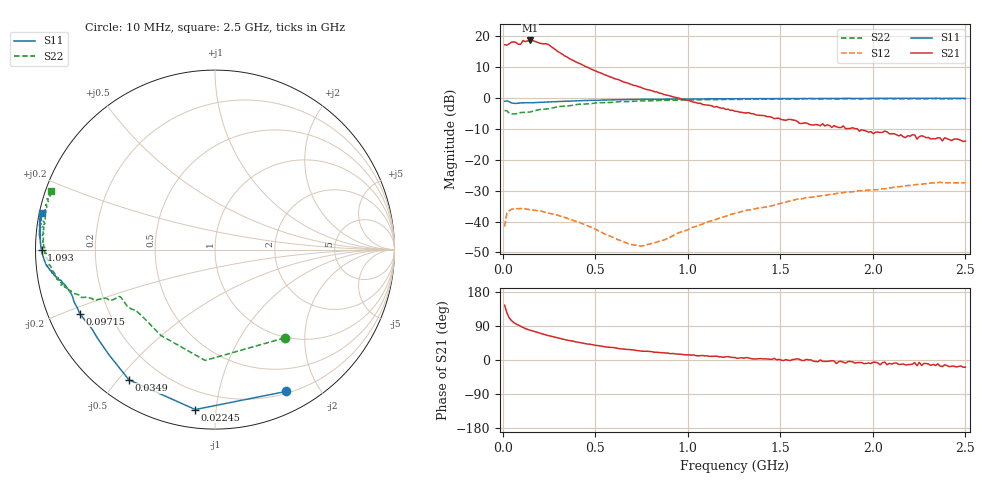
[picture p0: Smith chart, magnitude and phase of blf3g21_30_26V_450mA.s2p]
! Filename:  blf3g21_30_26V_450mA.s2p
! Philips part #: BLF3G21-30  !File created by 'SoftPlot Measurement Presentation'
! SoftPlot Measurement Presentation
! Start 10.000000000000 MHz  Stop 2.500000000000 GHz  Points 201
# MHZ S RI R 50
! S-Parameter data, F S11 S21 S12 S22
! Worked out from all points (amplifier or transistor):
!   201 points, 10 MHz to 2.5 GHz, reference 50 ohm
!   highest |S21| = 18.6 dB at 146.9 MHz (marker M1)
!   |S21| within 3 dB of that: start of sweep to 285.6 MHz
!   unconditionally stable (mu >= 1): 699.6 MHz to 710.6 MHz; 756.1 MHz to 793.7 MHz; 794.8 MHz to 815.4 MHz
!   at 420.9 MHz: K = 0.32, MSG = 25.7 dB, |S12| = -40.4 dB
!   at 1.255 GHz: K = 0.39, MSG = 16.5 dB, |S12| = -37.3 dB
!   at 2.5 GHz: K = -0.25, MSG = 6.7 dB, |S12| = -27.4 dB
!   S11 on the Smith chart (normalised r, x): 10 MHz: 0.22, -1.60; 22.45 MHz: 0.10, -0.88; 34.9 MHz: 0.09, -0.53; 97.15 MHz: 0.10, -0.22; 1.093 GHz: 0.02, -0.00; 2.5 GHz: 0.01, +0.10
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10  0.3972 -0.79  -5.935 4.204  0.00452 0.00698  0.3873 -0.4919
22.45  -0.1102 -0.891  -4.079 5.885  0.0111 0.00795  -0.0551 -0.6174
34.9  -0.48 -0.7255  -2.702 7.032  0.0138 0.0057  -0.3018 -0.4782
47.35  -0.5925 -0.5834  -1.922 7.77  0.0152 0.00433  -0.3757 -0.4019
59.8  -0.6537 -0.4952  -1.231 7.981  0.0158 0.00296  -0.418 -0.36
72.25  -0.6889 -0.4367  -0.7024 7.873  0.016 0.00194  -0.4411 -0.3392
84.7  -0.7222 -0.3963  -0.2546 7.384  0.0162 0.00108  -0.4665 -0.3308
97.15  -0.7534 -0.357  0.1897 7.403  0.0163 0.000406  -0.4895 -0.314
109.6  -0.7684 -0.3221  0.6112 8.493  0.0163 -0.000233  -0.5019 -0.2969
122.05  -0.7817 -0.2987  0.9998 8.089  0.016 -0.000987  -0.5145 -0.279
146.95  -0.7935 -0.2611  1.674 8.36  0.0154 -0.00181  -0.5319 -0.2614
246.55  -0.8374 -0.1938  3.185 6.609  0.0131 -0.00382  -0.6098 -0.2709
296.35  -0.8558 -0.1752  2.968 4.83  0.0121 -0.00409  -0.6628 -0.2831
333.7  -0.8688 -0.1669  2.842 3.882  0.0109 -0.00426  -0.6844 -0.2739
433.3  -0.8978 -0.1404  2.438 2.36  0.00847 -0.00348  -0.7504 -0.2574
632.5  -0.9345 -0.0952  1.677 0.958  0.00497 -0.000293  -0.8484 -0.2001
844.15  -0.954 -0.0494  1.132 0.4101  0.00281 0.0039  -0.9037 -0.1239
1093.15  -0.9663 -0.00312  0.762 0.1475  0.00112 0.00945  -0.9364 -0.0533
1255  -0.9712 0.0243  0.605 0.0693  0.000978 0.0136  -0.9496 -0.00331
1678.3  -0.9745 0.0911  0.3643 -0.0197  0.00409 0.0247  -0.9588 0.1107
2089.15  -0.976 0.1498  0.2604 -0.0401  0.0118 0.0329  -0.9484 0.2201
2500  -0.9631 0.2031  0.1896 -0.0655  0.0247 0.0346  -0.912 0.3243
